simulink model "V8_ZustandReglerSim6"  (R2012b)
settings: Solver=ode45  SolverMode=SingleTasking  StartTime=0.0  StopTime=10  RelTol=1e-3
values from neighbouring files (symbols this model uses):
  A = [1 1    [V8_1_ZustandRegler.m]    (also in V8_2_ZustandRegler.m; V8_2_ZustandRegler_dist.m; V8_3_ZustandRegler.m = [-1, 0, 0; V8_5_ZustandRegler.m)
  B = [0; 1]    [V8_1_ZustandRegler.m]    (also in V8_2_ZustandRegler.m; V8_2_ZustandRegler_dist.m; V8_3_ZustandRegler.m = [1; 0; 0]; V8_5_ZustandRegler.m)
  C = [1 0]    [V8_1_ZustandRegler.m]    (also in V8_2_ZustandRegler.m; V8_2_ZustandRegler_dist.m; V8_5_ZustandRegler.m; V8_7_ZustandRegler.m)
  F = place(A,B,pd)    [V8_1_ZustandRegler.m]    (also in V8_2_ZustandRegler.m; V8_2_ZustandRegler_dist.m; V8_3_ZustandRegler.m = S_c_n' * PA; V8_5_ZustandRegler.m)
  Fd = place(Ad,Bd,pdd)    [V8_7_ZustandRegler.m]
  Ts = 0.1    [V8_7_ZustandRegler.m]

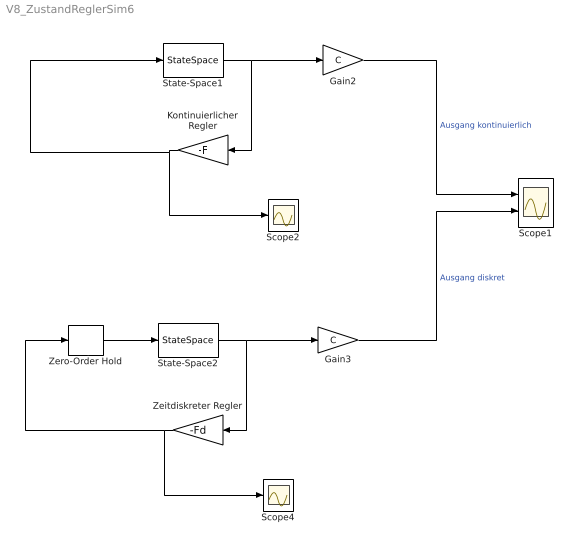
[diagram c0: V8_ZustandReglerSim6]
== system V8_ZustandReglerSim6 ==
  Gain2 : Gain  Gain=C  Multiplication=Matrix(K*u)
  Gain3 : Gain  Gain=C  Multiplication=Matrix(K*u)
  Kontinuierlicher Regler : Gain  Gain=-F  Multiplication=Matrix(K*u)
  Scope1 : Scope  NumInputPorts=2
  Scope2 : Scope
  Scope4 : Scope
  State-Space1 : StateSpace  A=A  B=B  C=eye(2)  D=[0; 0]  X0=[2; 2]
  State-Space2 : StateSpace  A=A  B=B  C=eye(2)  D=[0; 0]  X0=[2; 2]
  Zeitdiskreter Regler : Gain  Gain=-Fd  Multiplication=Matrix(K*u)
  Zero-Order Hold : ZeroOrderHold  SampleTime=Ts
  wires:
  State-Space1/1 -> Kontinuierlicher Regler/1, Gain2/1
  Kontinuierlicher Regler/1 -> State-Space1/1, Scope2/1
  Gain2/1 -> Scope1/1  "Ausgang kontinuierlich"
  State-Space2/1 -> Zeitdiskreter Regler/1, Gain3/1
  Zeitdiskreter Regler/1 -> Scope4/1, Zero-Order Hold/1
  Gain3/1 -> Scope1/2  "Ausgang diskret"
  Zero-Order Hold/1 -> State-Space2/1
